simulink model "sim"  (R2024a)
settings: Solver=VariableStepAuto  StartTime=0.0  StopTime=inf  RelTol=1e-3
undefined symbols (not defined in the file or in its folder): Fs, ip
libraries: ad936xlib x1, dspsrcs4 x1

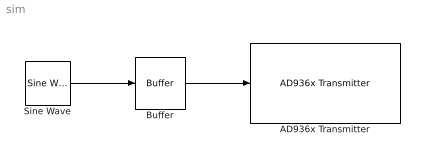
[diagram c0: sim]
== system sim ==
  AD936x Transmitter : ad936xlib/AD936x Transmitter  IPAddress=169.254.0.52  uri=ip:10.0.0.200  CenterFrequencySource=Dialog  CenterFrequency=2400000000  GainSource=Dialog  Gain=-10  ChannelMapping=1  BasebandSampleRate=60e6  UnderflowOutputPort=on  ShowAdvancedProperties=off  UseCustomFilter=off  filtPathRates=[737280000 11520000 3840000 1920000 960000 240000]  filtCoefficients="[-192 82 85 -215 228 -102 -110 290 -318 145 160 -426 471 -215 -238 633 -697 318 349 -923 1009 -457 -498 1309 -1423 640 693 -1812 1959 -876 -945 2458 -2647 1180 1268 -3290 3534 -1572 -1688 4375 -4698 2091 2247 -5836 6284 -2807 -3031 7918 -8588 3870 4225 -11182 12324 -5662 -6330 17255 -19735 9507 11312 -33568 43355 -25227 -42139 305542 305542 -42139 -25227 43355 -33568 11312 9507 -19735 17255 -6330 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"  filtCoefficientSize=128  filtDecimInterpFactor=4  filtGain=-12  filtRFBandwidth=18000000  filterConfigStruct=struct()  BypassUserLogic=off  DataSourceSelect=Input Port  DDSTone1Freq=5000  DDSTone2Freq=10000  DDSTone1Scale=0.5  DDSTone2Scale=0.25  DataTimeout=Inf  ENSMPinControlMode=None  BISTLoopbackMode=Disabled  BISTToneInject=Disabled  BISTSignalGen=PRBS  BISTToneFreq=Fs/32  BISTToneLevel=0
  Buffer : Buffer  N=9048  OutputFrames=off
  Sine Wave : dspsrcs4/Sine Wave  Amplitude=1  Frequency=100  Phase=0  SampleMode=Discrete  OutComplex=Complex  CompMethod=Trigonometric fcn  TableSize=Speed  SampleTime=1/1000  SamplesPerFrame=200  ResetState=Restart at time zero  OutputFrames=off  dataType=double  wordLen=16  udDataType=sfix(16)  fracBitsMode=Best precision  numFracBits=15  OutDataTypeStr=double  LastOutDataTypeStr=double
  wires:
  Sine Wave/1 -> Buffer/1
  Buffer/1 -> AD936x Transmitter/1
